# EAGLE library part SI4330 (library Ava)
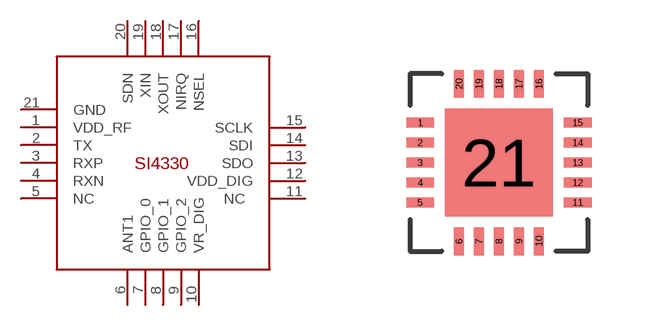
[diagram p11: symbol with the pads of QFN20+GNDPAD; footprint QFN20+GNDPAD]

Designator prefix -

## SI4330  [QFN20+GNDPAD]
1  VDD_RF
2  TX
3  RXP
4  RXN
5  NC
6  ANT1
7  GPIO_0
8  GPIO_1
9  GPIO_2
10  VR_DIG
11  NC
12  VDD_DIG
13  SDO
14  SDI
15  SCLK
16  NSEL
17  NIRQ
18  XOUT
19  XIN
20  SDN
21  GND

## Footprint QFN20+GNDPAD (pad centres in mm)
smd 0.7 x 0.25: 1 -1.97,1; 2 -1.97,0.5; 3 -1.97,0; 4 -1.97,-0.5; 5 -1.97,-1; 11 1.97,-1; 12 1.97,-0.5; 13 1.97,0; 14 1.97,0.5; 15 1.97,1
smd 0.25 x 0.7: 6 -1,-1.97; 7 -0.5,-1.97; 8 0,-1.97; 9 0.5,-1.97; 10 1,-1.97; 16 1,1.97; 17 0.5,1.97; 18 0,1.97; 19 -0.5,1.97; 20 -1,1.97
smd 2.7 x 2.7: 21 0,0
